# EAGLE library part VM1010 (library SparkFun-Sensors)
Vesper Technologies VM1010 The VM1010 is the world’s first ZeroPower ListeningTM piezoelectric MEMS microphone. It provides an ultra-low power always listening solution with a Wake on Sound mode that allows detection of voice activity.
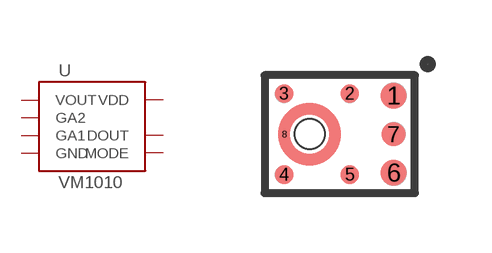
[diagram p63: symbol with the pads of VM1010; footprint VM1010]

Designator prefix -

## VM1010 (DIGIKEY_PART: 2022-1001-1-ND; MANU_PART: VM1010AA; PROD_ID: IC-15768)  [VM1010]
1  VOUT  out
2  GA2  in
3  GA1  in
4  GND  pwr
5  MODE  in
6  VDD  pwr
7  DOUT  out
8  GND  pwr

## Footprint VM1010 (pad centres in mm)
Vesper Technologies VM1010
smd 0.65 x 0.65: 1 1.35,0.965; 6 1.35,-0.965
smd 0.46 x 0.46: 2 0.25,1.015; 3 -1.39,1.015; 4 -1.39,-1.015; 5 0.25,-1.015
smd 0.6 x 0.6: 7 1.35,0
smd 0.25 x 0.25: 8 -1.38,0
hole 0.75 at -0.75,0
